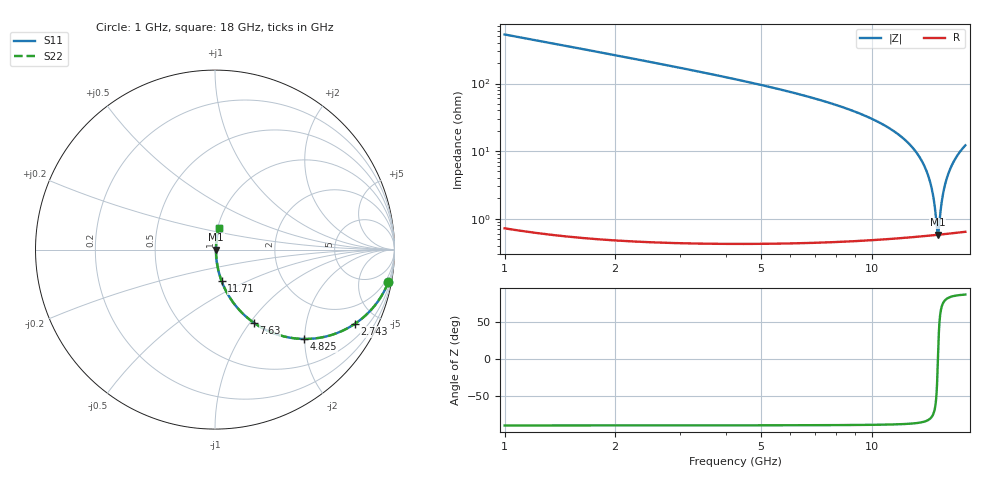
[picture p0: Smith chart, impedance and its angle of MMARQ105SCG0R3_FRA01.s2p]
! MMARQ105SCG0R3_FRA01  S-PARAMETER MODEL  ( Standard Model )
! Model Generated by TAIYO YUDEN Corporation (http://www.ty-top.com)
! Version 1.0
! TAIYO YUDEN Control No. 230906
! Copyright(c) 2023 TAIYO YUDEN CO.,LTD. All Rights Reserved.
! Product Description (link to TY-COMPAS)
! https://ds.yuden.co.jp/TYCOMPAS/or/detail?pn=MMARQ105SCG0R3BFRA01&u=M
! Products Name : Multilayer Ceramic Capacitors
! Characteristics :
!  Capacitance : 0.3 [pF] , Rated Voltage : 250 [V] , TCC : CG / C0G
!  Case Size : 1.0 x 0.5 / 0.039 x 0.02 [mm/inch] , Thickness : 0.5 / 0.02 [mm/inch]
!  (Conditions: Temperature = 25 [degC] , DC Bias Voltage = 0 [V])
! External Node Assignments :
!  1  o---| |---o  2
! GND o---------o GND
! Frequency Range : 1000MHz  -  18000MHz  [ 401 STEP ]
# MHZ S RI R 50
! Freq[MHz].  S11 Real  S11 Imag  S21 Real  S21 Imag  S12 Real  S12 Imag  S22 Real  S22 Imag
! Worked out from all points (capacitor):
!   401 points, 1 GHz to 18 GHz, reference 50 ohm
!   read as one part in series: C = 298 fF near 1.085 GHz
!   lowest |Z| = 578 mohm at 15.15 GHz (marker M1)
!   series resonance near 15.15 GHz, so ESL is about 370 pH
!   S11 on the Smith chart (normalised r, x): 1 GHz: 1, -11; 2.743 GHz: 1.01, -3.77; 4.825 GHz: 1.01, -1.99; 7.63 GHz: 1.01, -1.04; 11.71 GHz: 1.01, -0.37; 18 GHz: 1.01, +0.24
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1000  0.9656 -0.1816  0.0344 0.1816  0.0344 0.1816  0.9656 -0.1816
1765  0.8986 -0.301  0.1014 0.301  0.1014 0.301  0.8986 -0.301
2742.5  0.7795 -0.4134  0.2205 0.4134  0.2205 0.4134  0.7795 -0.4134
3847.5  0.6272 -0.4819  0.3728 0.4819  0.3728 0.4819  0.6272 -0.4819
4825  0.4971 -0.4979  0.5029 0.4979  0.5029 0.4979  0.4971 -0.4979
6695  0.2929 -0.4517  0.7071 0.4517  0.7071 0.4517  0.2929 -0.4517
7630  0.2162 -0.4074  0.7838 0.4074  0.7838 0.4074  0.2162 -0.4074
9500  0.1074 -0.3028  0.8926 0.3028  0.8926 0.3028  0.1074 -0.3028
11710  0.0371 -0.1757  0.9629 0.1757  0.9629 0.1757  0.0371 -0.1757
12347.5  0.0255 -0.1406  0.9745 0.1406  0.9745 0.1406  0.0255 -0.1406
13452.5  0.0123 -0.0824  0.9877 0.0824  0.9877 0.0824  0.0123 -0.0824
14217.5  0.00752 -0.0442  0.9925 0.0442  0.9925 0.0442  0.00752 -0.0442
14685  0.00612 -0.0217  0.9939 0.0217  0.9939 0.0217  0.00612 -0.0217
14855  0.00587 -0.0137  0.9941 0.0137  0.9941 0.0137  0.00587 -0.0137
15067.5  0.00574 -0.00386  0.9943 0.00386  0.9943 0.00386  0.00574 -0.00386
15152.5  0.00574 4.8e-05  0.9943 -4.8e-05  0.9943 -4.8e-05  0.00574 4.8e-05
15195  0.00576 0.002  0.9942 -0.002  0.9942 -0.002  0.00576 0.002
15577.5  0.00621 0.0193  0.9938 -0.0193  0.9938 -0.0193  0.00621 0.0193
15790  0.0067 0.0287  0.9933 -0.0287  0.9933 -0.0287  0.0067 0.0287
16087.5  0.00768 0.0416  0.9923 -0.0416  0.9923 -0.0416  0.00768 0.0416
16895  0.0119 0.0754  0.9881 -0.0754  0.9881 -0.0754  0.0119 0.0754
18000  0.0207 0.1184  0.9793 -0.1184  0.9793 -0.1184  0.0207 0.1184
